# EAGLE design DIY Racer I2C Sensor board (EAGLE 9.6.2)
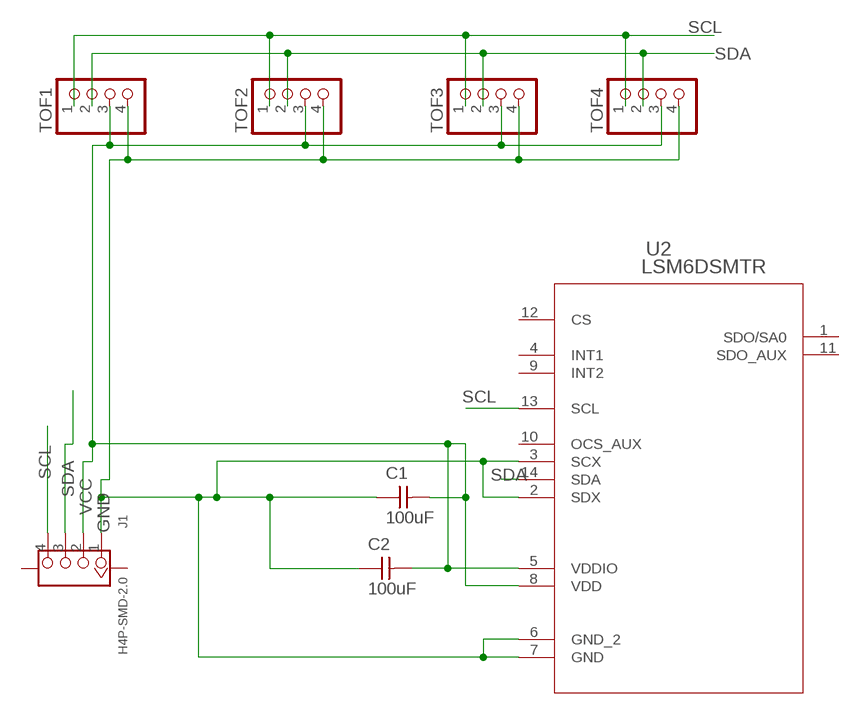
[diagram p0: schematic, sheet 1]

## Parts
C1  100uF  CAP_UNPOLARIZED  [C1206]
C2  100uF  CAP_UNPOLARIZED  [C1206]
J1  H4P-SMD-2.0  GROVE-CONNECTOR-SMD(4+2P-2.0)  [HW4-SMD-2.0]
TOF1  PINHD-1X04_2.54-SMD  [1X04SMD]
TOF2  PINHD-1X04_2.54-SMD  [1X04SMD]
TOF3  PINHD-1X04_2.54-SMD  [1X04SMD]
TOF4  PINHD-1X04_2.54-SMD  [1X04SMD]
U2  LSM6DSMTR  [LGA-14L_2P5X3X0P83_STM]

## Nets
GND: C1.1 C2.1 J1.1 TOF1.4 TOF2.4 TOF3.4 TOF4.4 U2.2(SDX) U2.3(SCX) U2.6(GND_2) U2.7(GND)
SCL: J1.4 TOF1.1 TOF2.1 TOF3.1 TOF4.1 U2.13(SCL)
SDA: J1.3 TOF1.2 TOF2.2 TOF3.2 TOF4.2 U2.14(SDA)
VCC: C1.2 C2.2 J1.2 TOF1.3 TOF2.3 TOF3.3 TOF4.3 U2.5(VDDIO) U2.8(VDD)
Unconnected: J1.SS1 J1.SS2 U2.1(SDO/SA0) U2.4(INT1) U2.9(INT2) U2.10(OCS_AUX) U2.11(SDO_AUX) U2.12(CS)

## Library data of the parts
C1 C2 = fab:CAP_UNPOLARIZED
J1 = OPL_Connector:GROVE-CONNECTOR-SMD(4+2P-2.0): 320110030
TOF1-TOF4 = pinhead-2:PINHD-1X04: PIN HEADER
U2 = LSM6DSMTR:LSM6DSMTR; BUILT_BY: EMA_Cory; COPYRIGHT: Copyright (C) 2018 Accelerated Designs. All rights reserved; DATASHEET: https://www.st.com/content/ccc/resource/technical/document/datasheet/76/27/cf/88/c5/03/42/6b/DM00218116.pdf/files/DM00218116.pdf/jcr:content/translations/en.DM00218116.pdf; MANUFACTURER_PART_NUMBER: LSM6DSMTR; SOURCELIBRARY: Updates_to_database_2020-11-03; VENDOR: STMicroelectronics

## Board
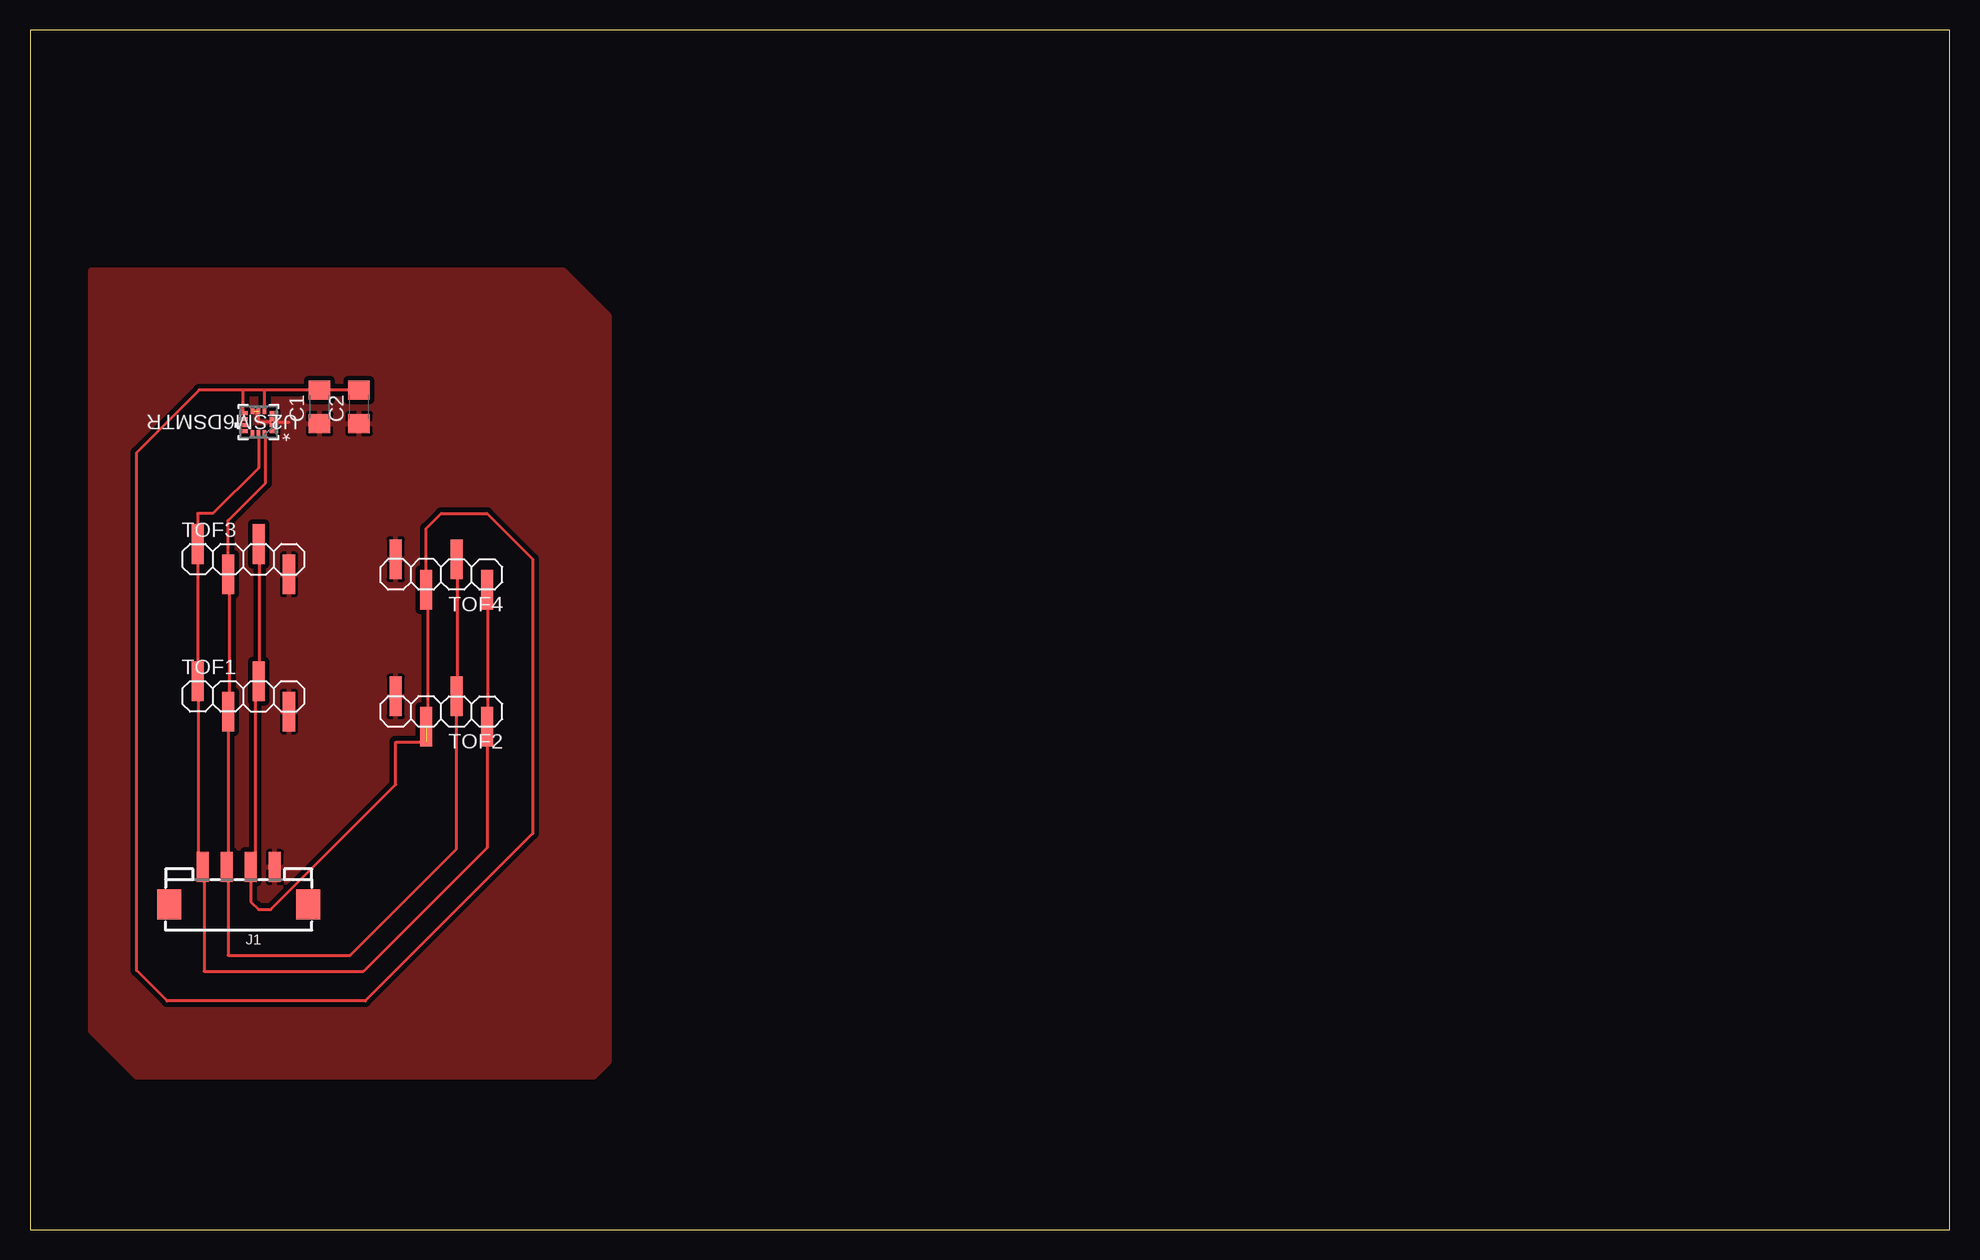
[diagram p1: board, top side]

Size 160 x 100 mm. Coordinates in mm from the lower left corner, seen from the top.
Outline: 0,0 160,0 160,100 0,100 0,0
Copper layers (1*16): Top 0.035mm / dielectric 1.5mm / Bottom 0.035mm
Design rules "default *": minimum track width 0.25mm, minimum drill 0.35mm, track to track 0.4mm, track to pad 0.19mm, pad to pad 0.19mm, via to via 0.4mm, smd to smd 0.19mm, copper to edge 40mil, drill to drill 6mil, minimum pad ring 10mil, minimum via ring 8mil, stop-mask expansion 4mil, vias tented up to drill 0mil, thermal gap 10mil

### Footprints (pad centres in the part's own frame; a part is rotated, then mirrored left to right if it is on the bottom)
C1206 = smd 1.6 x 1.8: 1 -1.4,0; 2 1.4,0
HW4-SMD-2.0 = smd 1 x 2.5: 1 -3,0; 2 -1,0; 3 1,0; 4 3,0 | smd 2 x 2.5: SS1 -5.8,3.123; SS2 5.8,3.123
1X04SMD = smd 1.016 x 3.302: 1 -1.27,1.27; 2 1.27,-1.27; 3 3.81,1.27; 4 6.35,-1.27
LGA-14L_2P5X3X0P83_STM = smd 0.533 x 0.305: 1 -1.181,0.75; 2 -1.181,0.25; 3 -1.181,-0.25; 4 -1.181,-0.75; 8 1.181,-0.75; 9 1.181,-0.25; 10 1.181,0.25; 11 1.181,0.75 | smd 0.305 x 0.533: 5 -0.5,-0.927; 6 0,-0.927; 7 0.5,-0.927; 12 0.5,0.927; 13 0,0.927; 14 -0.5,0.927

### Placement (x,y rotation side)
C1  24.13,68.58 90 top
C2  27.43,68.58 90 top
J1  17.4,30.23 180 top
TOF1  15.24,44.45 0 top
TOF2  36.83,43.18 180 top
TOF3  15.24,55.88 0 top
TOF4  36.83,54.61 180 top
U2  19.05,67.31 180 top

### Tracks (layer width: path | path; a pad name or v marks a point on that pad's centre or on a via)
GND  (1 unrouted)
  Top 0.25: 20.23,67.1 20.25,67.12 U2.2 | U2.3 20.25,67.5 20.23,67.5 | U2.3 20.48,67.31 21.59,67.31 | U2.3 19.98,67.31 19.05,67.31 19.05,67.77 18.89,67.92 18.89,68.21 18.87,68.24 18.65,68.24
  pour Top: 5.08,80.01 44.45,80.01 48.26,76.2 48.26,13.97 46.99,12.7 8.89,12.7 6.35,15.24 5.08,16.51
SCL
  Top 0.25: TOF4.1 38.12,53.25 38.12,42 TOF2.1 38.1,31.82 27.81,21.52 14.5,21.52 14.5,30.12 J1.4 14,30.62 14,45.62 TOF1.1 14,45.75 14,57.12 TOF3.1 13.97,59.69 15.24,59.69 19.05,63.5 U2.13
SDA
  Top 0.25: U2.14 19.62,66.38 19.62,62.23 16.51,59.12 TOF3.2 16.62,54.5 16.62,43.25 TOF1.2 16.5,43.12 16.5,30.25 J1.3 16.51,30.11 16.51,22.86 26.67,22.86 35.56,31.75 35.56,41.91 35.56,43.18 TOF2.2 | 35.5,44.38 TOF2.2 | TOF4.2 35.62,55.88 35.62,44.5 TOF2.2
VCC  (1 unrouted)
  Top 0.25: TOF2.3 33.12,42 33.12,53.25 TOF4.3 | 33,53.38 TOF4.3 | 19,57.25 TOF3.3 19.12,57.12 19.12,45.75 TOF1.3 19,45.62 18.75,45.38 18.75,30.5 18.5,30.25 J1.2 18.4,27.32 19.05,26.67 20.07,26.67 30.48,37.08 30.48,40.64 33.02,40.64 | TOF4.3 33.02,58.42 34.29,59.69 38.1,59.69 41.91,55.88 41.91,33.02 27.94,19.05 11.43,19.05 8.89,21.59 8.89,64.77 14.1,69.98 17.78,69.98 | C2.2 C1.2 19.56,69.98 | 19.56,69.98 17.78,69.98 | U2.8 17.78,68.15 17.78,69.98 | U2.5 19.55,69.97 19.56,69.98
